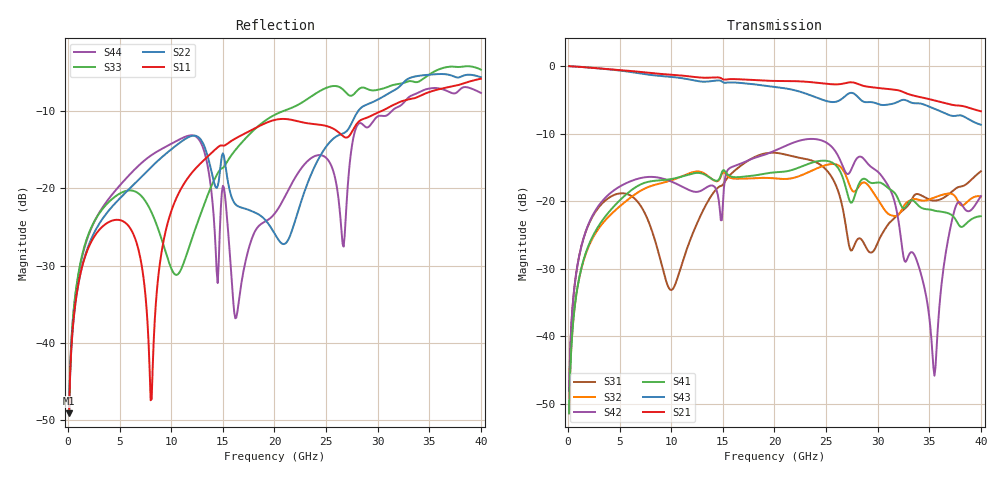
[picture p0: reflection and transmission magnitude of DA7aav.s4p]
! ADC12DJ2700AAV, ADC12DJ3200AAV, ADC08DJ3200AAV
! 144 pin AAV package
! Texas Instruments 4/21/2021
! Single-ended  S-parameters
! PORT#  PORT_NAME  NET_NAME
! PORT1:  DAxN.DIEBUMP DAxN
! PORT2:  DAxN.BGA  DAxN
! PORT3:  DAxP.DIEBUMP DAxP
! PORT4:  DAxP.BGA  DAxP
! Touchstone Ver. 1.0
! Number of ports is 4
# Hz	S	MA	R	50.000000
! SCATTERING PARAMETERS  :
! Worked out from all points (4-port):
!   400 points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, 100 MHz to 40 GHz, reference 50 ohm
!   strongest paths, dB at 100 MHz, 10.1 GHz, 20.1 GHz, 30.1 GHz, 40 GHz:
!     S21: 0.0, -1.3, -2.2, -3.3, -6.7
!     S43: 0.0, -1.6, -3.1, -5.6, -8.7
!     S41: -51.4, -16.7, -15.7, -17.2, -22.2
!     S42: -48.2, -17.2, -12.5, -15.8, -19.3
!     S32: -51.4, -16.9, -16.6, -19.9, -19.3
!     S31: -48.2, -33.1, -12.8, -25.8, -15.6
!   lowest |S11| = -49.2 dB at 100 MHz (marker M1), VSWR 1.01, Z = 50.2 + j0.311 ohm
!   |S11| at or under -10 dB: start of sweep to 30.31 GHz
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1e8  0.003485 62.9  0.9982 -1.3  0.003905 85.3  0.002685 -95.6
     0.9982 -1.3  0.003477 62.6  0.002685 -95.7  0.003902 85.7
     0.003905 85.3  0.002685 -95.7  0.003729 66.8  0.9983 -1.3
     0.002685 -95.6  0.003902 85.7  0.9983 -1.3  0.00371 67.0
7e9  0.03536 -48.9  0.9047 -82.2  0.0931 -45.4  0.1326 150.6
     0.9047 -82.2  0.1171 -24.6  0.119 158.1  0.148 4.0
     0.0931 -45.4  0.119 158.1  0.09069 -66.8  0.8813 -80.1
     0.1326 150.6  0.148 4.0  0.8813 -80.1  0.144 -5.7
8.1e9  0.004308 34.6  0.8863 -94.2  0.06111 -74.8  0.1406 131.9
       0.8863 -94.2  0.1386 -37.0  0.1299 141.7  0.1512 -10.0
       0.06111 -74.8  0.1299 141.7  0.06964 -98.4  0.8578 -91.4
       0.1406 131.9  0.1512 -10.0  0.8578 -91.4  0.1647 -20.5
1.62e10  0.2105 -21.7  0.8006 178.8  0.1697 63.7  0.1503 24.0
         0.8006 178.8  0.07917 -146.4  0.1466 34.4  0.1828 78.5
         0.1697 63.7  0.1466 34.4  0.1771 22.5  0.7552 -174.0
         0.1503 24.0  0.1828 78.5  0.7552 -174.0  0.01438 79.7
2.34e10  0.2634 -89.5  0.762 99.1  0.202 -28.6  0.1903 -63.3
         0.762 99.1  0.1166 27.7  0.1652 -41.1  0.2887 -1.8
         0.202 -28.6  0.1652 -41.1  0.3884 -50.3  0.6115 108.2
         0.1903 -63.3  0.2887 -1.8  0.6115 108.2  0.1545 -31.2
3.55e10  0.4322 178.3  0.5562 -42.5  0.101 37.7  0.08497 144.3
         0.5562 -42.5  0.55 -92.8  0.1065 -172.3  0.0051 12.5
         0.101 37.7  0.1065 -172.3  0.5742 -139.5  0.4832 -14.7
         0.08497 144.3  0.0051 12.5  0.4832 -14.7  0.4484 -75.9
4e10  0.515 93.6  0.4627 -91.6  0.1663 16.1  0.07732 104.9
      0.4627 -91.6  0.5265 -119.6  0.1082 129.0  0.1089 45.1
      0.1663 16.1  0.1082 129.0  0.59 159.5  0.3677 -57.3
      0.07732 104.9  0.1089 45.1  0.3677 -57.3  0.4164 -105.4
